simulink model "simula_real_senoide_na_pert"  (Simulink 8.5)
settings: Solver=ode45  StartTime=0.0  StopTime=tf  FixedStep=dt  RelTol=1e-6
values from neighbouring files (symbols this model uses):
  Areal = [zeros(n2,n2) eye(n2); -Pinv*R -Pinv*Q]    [mod_estados_real.m]
  Breal = [zeros(n2,1); Pinv*U]    [mod_estados_real.m]
  Creal = zeros(1,2*n2)    [mod_estados_real.m]
  denK = [1/6 1]    [princi_JL_incerto_prefilt_2a_ordem.m]
  Dreal = 0    [mod_estados_real.m]
  numK = 2.5    [princi_JL_incerto_prefilt_2a_ordem.m]
undefined symbols (not defined in the file or in its folder): w0_pert

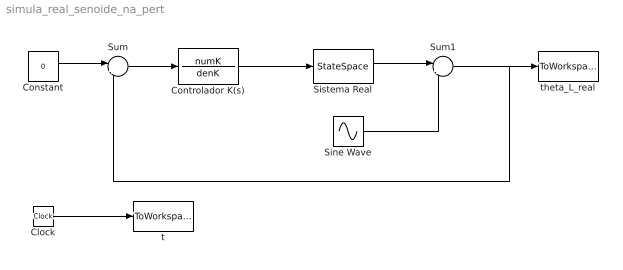
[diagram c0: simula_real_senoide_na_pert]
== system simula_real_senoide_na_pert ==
  Clock : Clock
  Constant : Constant  Value=0
  Controlador K(s) : TransferFcn  Numerator=numK  Denominator=denK
  Sine Wave : Sin  Frequency=w0_pert  SampleTime=0
  Sistema Real : StateSpace  A=Areal  B=Breal  C=Creal  D=Dreal  X0=0
  Sum : Sum  Inputs=|+-
  Sum1 : Sum  Inputs=|++
  t : ToWorkspace  VariableName=t  SampleTime=-1
  theta_L_real : ToWorkspace  VariableName=theta_L_real  SampleTime=-1
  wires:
  Sum/1 -> Controlador K(s)/1
  Constant/1 -> Sum/1
  Clock/1 -> t/1
  Controlador K(s)/1 -> Sistema Real/1
  Sistema Real/1 -> Sum1/1
  Sum1/1 -> Sum/2, theta_L_real/1
  Sine Wave/1 -> Sum1/2
